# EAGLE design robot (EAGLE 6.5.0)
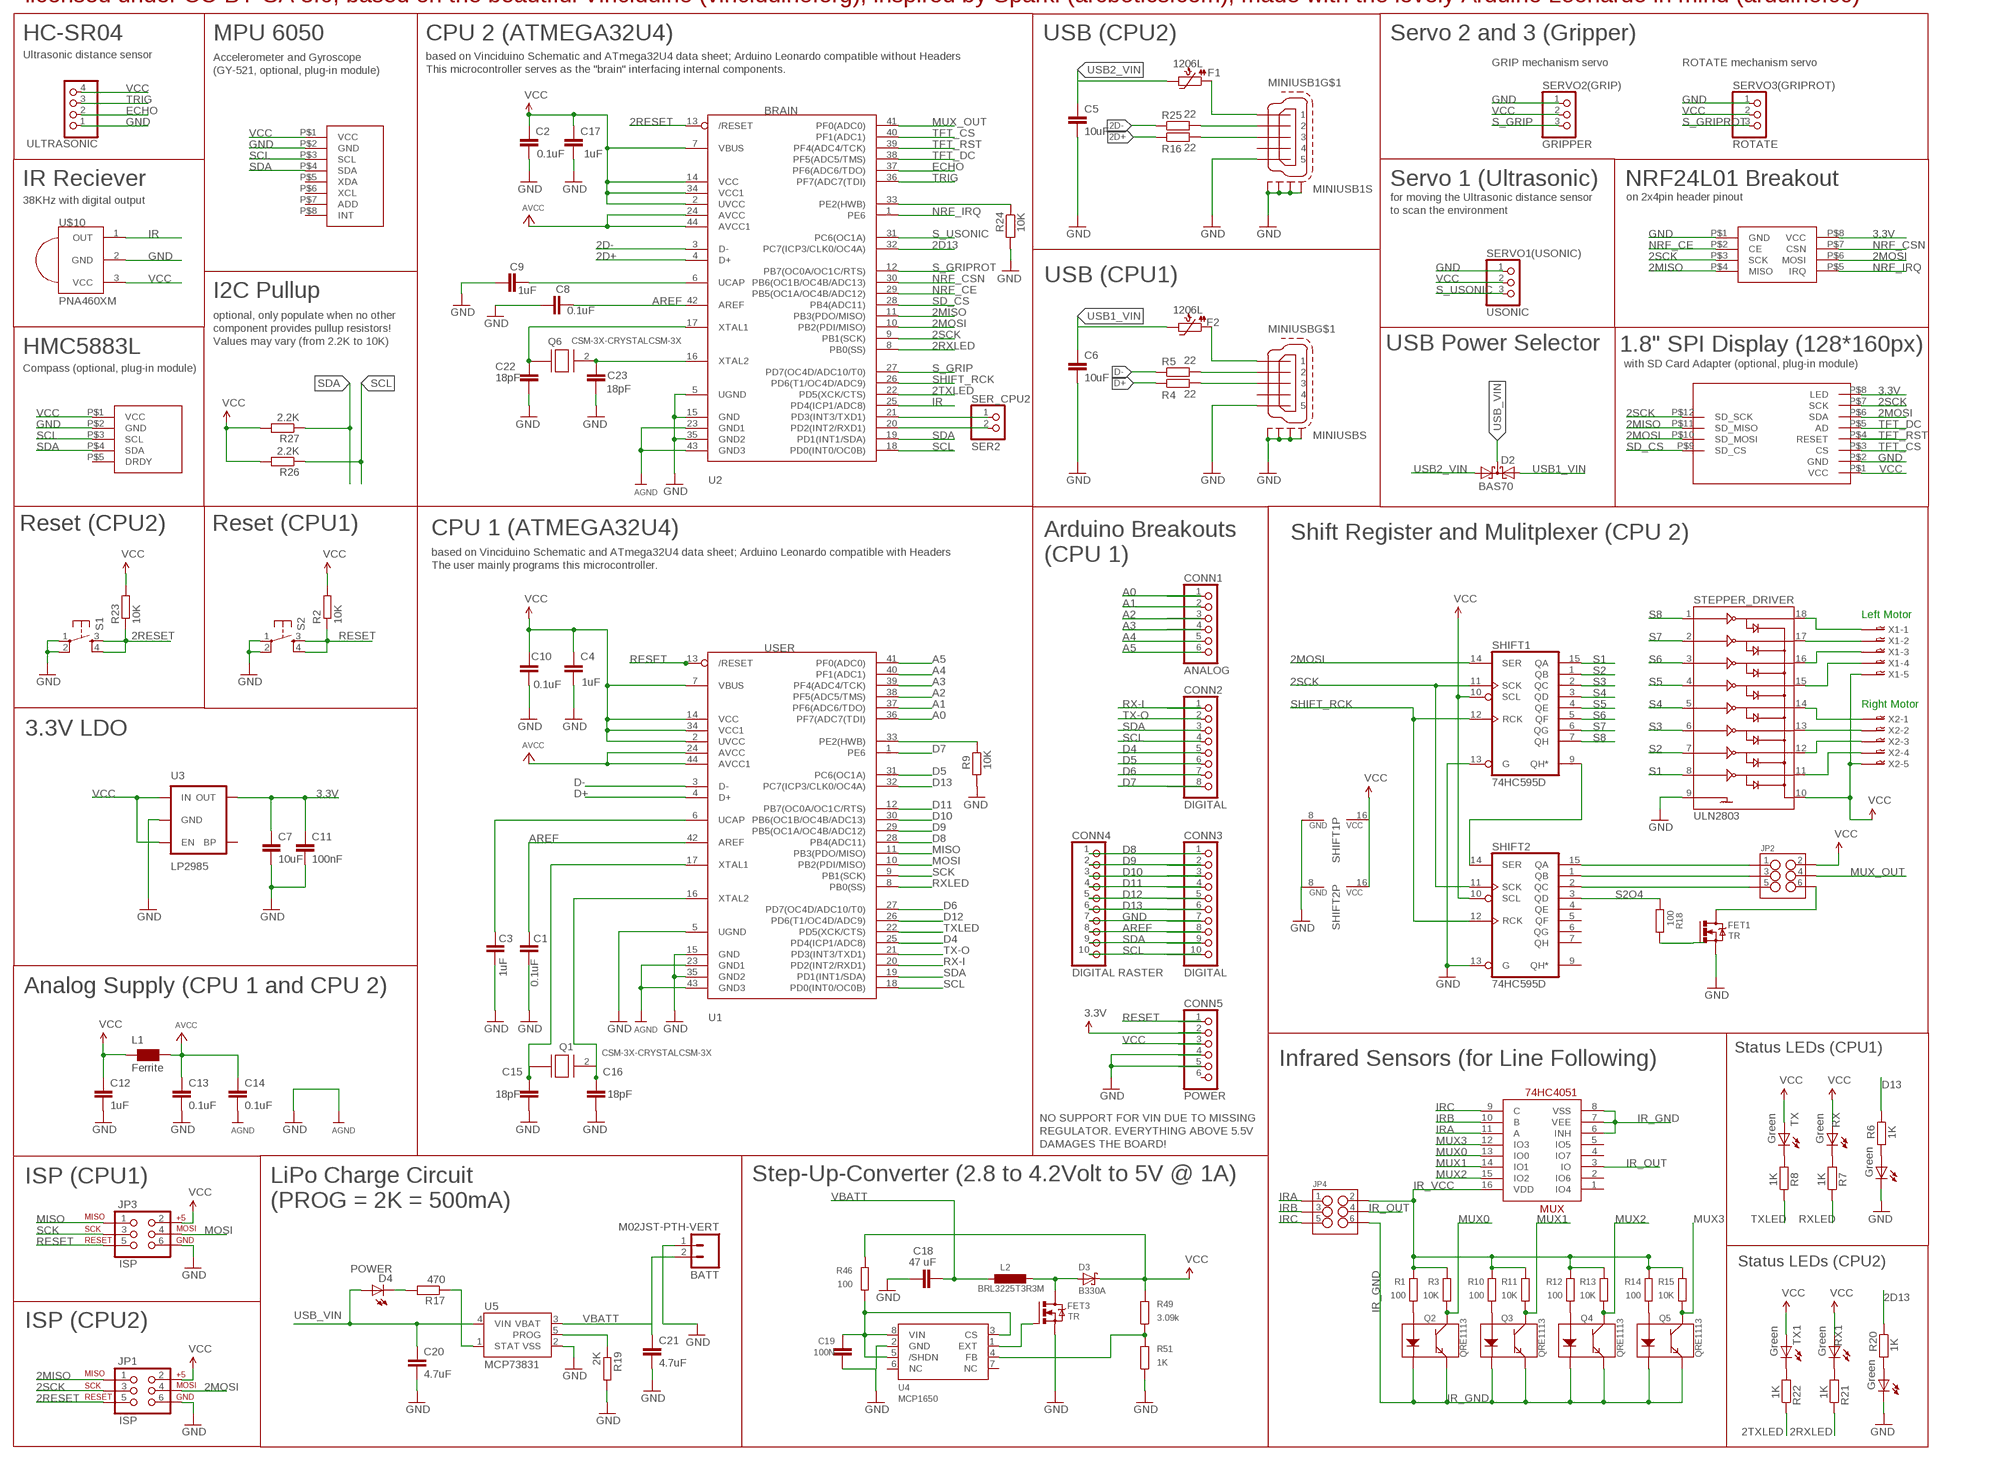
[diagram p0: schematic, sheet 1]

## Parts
BATT  M02JST-PTH-VERT  [JST-2-PTH-VERT]
C1  0.1uF  C-EUC1206  [C1206]
C2  0.1uF  C-EUC1206  [C1206]
C3  1uF  C-EUC1206  [C1206]
C4  1uF  C-EUC1206  [C1206]
C5  10uF  C-EUC1206  [C1206]
C6  10uF  C-EUC1206  [C1206]
C7  10uF  C-EUC1206  [C1206]
C8  0.1uF  C-EUC1206  [C1206]
C9  1uF  C-EUC1206  [C1206]
C10  0.1uF  C-EUC1206  [C1206]
C11  100nF  C-EUC1206  [C1206]
C12  1uF  C-EUC1206  [C1206]
C13  0.1uF  C-EUC1206  [C1206]
C14  0.1uF  C-EUC1206  [C1206]
C15  18pF  C-EUC1206  [C1206]
C16  18pF  C-EUC1206  [C1206]
C17  1uF  C-EUC1206  [C1206]
C18  47 uF  C-EUC1206  [C1206]
C19  100N  C-EUC1206  [C1206]
C20  4.7uF  C-EUC1206  [C1206]
C21  4.7uF  C-EUC1206  [C1206]
C22  18pF  C-EUC1206  [C1206]
C23  18pF  C-EUC1206  [C1206]
CONN1  ANALOG  PINHD-1X6B  [1X06-BIG]
CONN2  DIGITAL  PINHD-1X8BIG  [1X08-BIG]
CONN3  DIGITAL  PINHD-1X10  [1X10-BIG]
CONN4  DIGITAL RASTER  PINHD-1X10  [1X10-BIG]
CONN5  POWER  PINHD-1X6B  [1X06-BIG]
D2  BAS70  BAS70-05  [SOT23]
D3  B330A  [SMA]
D4  POWER  LED1206  [LED-1206]
D13  Green  LED1206  [LED-1206]
D13_2  Green  LED1206  [LED-1206]
F1  1206L  PTC1206_L  [1206_PTC]
F2  1206L  PTC1206_L  [1206_PTC]
FET1  TR  IRLML2502TR  [MICRO3]
FET3  TR  IRLML2502TR  [MICRO3]
JP1  ISP  AVR_SPI_PRG_6PTH  [2X3]
JP2  M03X22X3_SILK_SM  [2X3]
JP3  ISP  AVR_SPI_PRG_6PTH  [2X3]
JP4  M03X22X3_SILK_SM  [2X3]
L1  Ferrite  WE-CBF_1206W  [1206W]
L2  BRL3225T3R3M  L-EUL3225P  [L3225P]
MINIUSB  MINI-USB-SCHIELD-32005-201  [32005-201]
MINIUSB1  MINI-USB-SCHIELD-32005-201  [32005-201]
MUX  74HC4051  74HC4051_MUX  [SO16]
Q1  CSM-3X-CRYSTALCSM-3X  [CSM-3X]
Q2  QRE1113  [QRE1113]
Q3  QRE1113  [QRE1113]
Q4  QRE1113  [QRE1113]
Q5  QRE1113  [QRE1113]
Q6  CSM-3X-CRYSTALCSM-3X  [CSM-3X]
R1  100  R-EU_R1206  [R1206]
R2  10K  R-EU_R1206  [R1206]
R3  10K  R-EU_R1206  [R1206]
R4  22  R-EU_R1206  [R1206]
R5  22  R-EU_R1206  [R1206]
R6  1K  R-EU_R1206  [R1206]
R7  1K  R-EU_R1206  [R1206]
R8  1K  R-EU_R1206  [R1206]
R9  10K  R-EU_R1206  [R1206]
R10  100  R-EU_R1206  [R1206]
R11  10K  R-EU_R1206  [R1206]
R12  100  R-EU_R1206  [R1206]
R13  10K  R-EU_R1206  [R1206]
R14  100  R-EU_R1206  [R1206]
R15  10K  R-EU_R1206  [R1206]
R16  22  R-EU_R1206  [R1206]
R17  470  R-EU_R1206  [R1206]
R18  100  R-EU_R1206  [R1206]
R19  2K  R-EU_R1206  [R1206]
R20  1K  R-EU_R1206  [R1206]
R21  1K  R-EU_R1206  [R1206]
R22  1K  R-EU_R1206  [R1206]
R23  10K  R-EU_R1206  [R1206]
R24  10K  R-EU_R1206  [R1206]
R25  22  R-EU_R1206  [R1206]
R26  2.2K  R-EU_R1206  [R1206]
R27  2.2K  R-EU_R1206  [R1206]
R46  100  R-EU_R1206  [R1206]
R49  3.09k  R-EU_R1206  [R1206]
R51  1K  R-EU_R1206  [R1206]
RX  Green  LED1206  [LED-1206]
RX1  Green  LED1206  [LED-1206]
S1  Reset  TAC_SWITCHSMD  [TACTILE_SWITCH_SMD]
S2  Reset  TAC_SWITCHSMD  [TACTILE_SWITCH_SMD]
SER_CPU2  SER2  PINHD-1X2  [1X02]
SERVO1(USONIC)  USONIC  PINHD-1X3  [1X03]
SERVO2(GRIP)  GRIPPER  PINHD-1X3  [1X03]
SERVO3(GRIPROT)  ROTATE  PINHD-1X3  [1X03]
SHIFT1  74HC595D  [SO16]
SHIFT2  74HC595D  [SO16]
STEPPER_DRIVER  ULN2803  ULN2803SOIC  [SO018]
TX  Green  LED1206  [LED-1206]
TX1  Green  LED1206  [LED-1206]
U1  USER  ATMEGA32U4-AU  [TQFP44]
U2  BRAIN  ATMEGA32U4-AU  [TQFP44]
U3  LP2985  V_REG_LDOSMD  [SOT23-5@1]
U4  MCP1650  [MSOP8]
U5  MCP73831  MCP73831SMD  [SOT23-5]
U$2  1.8TFT+SD  [1.8TFTSD]
U$3  GY-521  [GY-521]
U$4  HMC5883L  [HMC5883L]
U$5  NRF24L01+  [NRF24L01+]
U$10  PNA460XM  [PNA460XM]
ULTRASONIC  PINHD-1X4  [1X04]
X1  05-JST-B5B-XH-A  [B5B-XH]
X2  05-JST-B5B-XH-A  [B5B-XH]

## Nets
2D13: R20.1 U2.32(PC7(ICP3/CLK0/OC4A))
2D+: R16.1 U2.4(D+)
2D-: R25.1 U2.3(D-)
2MISO: JP1.1 U2.11(PB3(PDO/MISO)) U$2.P$11(SD_MISO) U$5.P$4(MISO)
2MOSI: JP1.4 SHIFT1.14(SER) U2.10(PB2(PDI/MISO)) U$2.P$6(SDA) U$2.P$10(SD_MOSI) U$5.P$6(MOSI)
2RESET: JP1.5 R23.1 S1.3 S1.4 U2.13(/RESET)
2RXLED: R21.1 U2.8(PB0(SS))
2SCK: JP1.3 SHIFT1.11(SCK) SHIFT2.11(SCK) U2.9(PB1(SCK)) U$2.P$7(SCK) U$2.P$12(SD_SCK) U$5.P$3(SCK)
2TXLED: R22.1 U2.22(PD5(XCK/CTS))
2XTAL1: C22.1 Q6.1 U2.17(XTAL1)
2XTAL2: C23.1 Q6.2 U2.16(XTAL2)
3.3V: C7.1 C11.1 CONN5.2 U3.5(OUT) U$2.P$8(LED) U$5.P$8(VCC)
A0: CONN1.1 U1.36(PF7(ADC7(TDI))
A1: CONN1.2 U1.37(PF6(ADC6/TDO))
A2: CONN1.3 U1.38(PF5(ADC5/TMS))
A3: CONN1.4 U1.39(PF4(ADC4/TCK))
A4: CONN1.5 U1.40(PF1(ADC1))
A5: CONN1.6 U1.41(PF0(ADC0))
AREF: C1.2 C8.2 CONN3.8 CONN4.8 U1.42(AREF) U2.42(AREF)
AVCC: C13.1 C14.1 L1.2 U1.24(AVCC) U1.44(AVCC1) U2.24(AVCC) U2.44(AVCC1)
D4: CONN2.5 U1.25(PD4(ICP1/ADC8))
D5: CONN2.6 U1.31(PC6(OC1A))
D6: CONN2.7 U1.27(PD7(OC4D/ADC10/T0))
D7: CONN2.8 U1.1(PE6)
D8: CONN3.1 CONN4.1 U1.28(PB4(ADC11))
D9: CONN3.2 CONN4.2 U1.29(PB5(OC1A/OC4B/ADC12))
D10: CONN3.3 CONN4.3 U1.30(PB6(OC1B/OC4B/ADC13))
D11: CONN3.4 CONN4.4 U1.12(PB7(OC0A/OC1C/RTS))
D12: CONN3.5 CONN4.5 U1.26(PD6(T1/OC4D/ADC9))
D13: CONN3.6 CONN4.6 R6.1 U1.32(PC7(ICP3/CLK0/OC4A))
D+: R4.1 U1.4(D+)
D-: R5.1 U1.3(D-)
ECHO: U2.37(PF6(ADC6/TDO)) ULTRASONIC.2
GND: BATT.1 C1.1 C2.2 C3.2 C4.2 C5.2 C6.2 C7.2 C8.1 C9.2 C10.2 C11.2 C12.2 C13.2 C14.2 C15.2 C16.2 C17.2 C18.1 C19.2 C20.2 C21.2 C22.2 C23.2 CONN3.7 CONN4.7 CONN5.4 CONN5.5 D13.C D13_2.C FET1.2(S) FET3.2(S) JP1.6 JP3.6 MINIUSB1.5 MINIUSB1.M1(S:S1) MINIUSB1.M2(S:S2) MINIUSB1.M3(S:S3) MINIUSB1.M4(S:S4) MINIUSB.5 MINIUSB.M1(S:S1) MINIUSB.M2(S:S2) MINIUSB.M3(S:S3) MINIUSB.M4(S:S4) R9.2 R19.2 R24.2 R51.1 S1.1 S1.2 S2.1 S2.2 SERVO1(USONIC).1 SERVO2(GRIP).1 SERVO3(GRIPROT).1 SHIFT1.8(GND) SHIFT1.13(G) SHIFT2.8(GND) SHIFT2.13(G) STEPPER_DRIVER.9 U1.5(UGND) U1.15(GND) U1.23(GND1) U1.35(GND2) U1.43(GND3) U2.5(UGND) U2.15(GND) U2.23(GND1) U2.35(GND2) U2.43(GND3) U3.2(GND) U4.2(GND) U5.2(VSS) U$2.P$2(GND) U$3.P$2(GND) U$4.P$2(GND) U$5.P$1(GND) U$10.2(GND) ULTRASONIC.1 ; supply symbol labelled AGND
IR: U2.25(PD4(ICP1/ADC8)) U$10.1(OUT)
IR_GND: JP4.6 MUX.6(INH) MUX.7(VEE) MUX.8(VSS) Q2.2(K) Q2.4(E) Q3.2(K) Q3.4(E) Q4.2(K) Q4.4(E) Q5.2(K) Q5.4(E)
IR_OUT: JP4.4 MUX.3(IO)
IR_VCC: JP4.2 MUX.16(VDD) R1.2 R3.2 R10.2 R11.2 R12.2 R13.2 R14.2 R15.2
IRA: JP4.1 MUX.11(A)
IRB: JP4.3 MUX.10(B)
IRC: JP4.5 MUX.9(C)
MISO: JP3.1 U1.11(PB3(PDO/MISO))
MOSI: JP3.4 U1.10(PB2(PDI/MISO))
MUX0: MUX.13(IO0) Q2.3(C) R3.1
MUX1: MUX.14(IO1) Q3.3(C) R11.1
MUX2: MUX.15(IO2) Q4.3(C) R13.1
MUX3: MUX.12(IO3) Q5.3(C) R15.1
MUX_OUT: JP2.4 U2.41(PF0(ADC0))
N$1: R8.2 TX.C
N$2: MINIUSB.2 R5.2
N$3: SER_CPU2.1 U2.21(PD3(INT3/TXD1))
N$4: SER_CPU2.2 U2.20(PD2(INT2/RXD1))
N$5: MINIUSB.3 R4.2
N$6: R9.1 U1.33(PE2(HWB))
N$7: D13.A R6.2
N$8: C9.1 U2.6(UCAP)
N$9: R7.2 RX.C
N$10: Q2.1(A) R1.1
N$11: Q3.1(A) R10.1
N$12: Q4.1(A) R12.1
N$13: F2.1 MINIUSB.1
N$14: Q5.1(A) R14.1
N$15: C3.1 U1.6(UCAP)
N$16: FET1.1(G) R18.2
N$17: R24.1 U2.33(PE2(HWB))
N$18: F1.1 MINIUSB1.1
N$19: FET3.1(G) U4.1(EXT)
N$20: R19.1 U5.5(PROG)
N$21: R17.1 U5.1(STAT)
N$22: D4.C R17.2
N$23: R49.1 R51.2 U4.4(FB)
N$24: D3.A FET3.3(D) L2.2
N$25: C19.1 R46.1 U4.3(CS) U4.5(/SHDN) U4.8(VIN)
N$26: STEPPER_DRIVER.11 X2.P$4
N$27: STEPPER_DRIVER.12 X2.P$3
N$28: STEPPER_DRIVER.13 X2.P$2
N$29: STEPPER_DRIVER.14 X2.P$1
N$30: STEPPER_DRIVER.15 X1.P$4
N$31: STEPPER_DRIVER.16 X1.P$3
N$32: STEPPER_DRIVER.17 X1.P$2
N$33: STEPPER_DRIVER.18 X1.P$1
N$34: D13_2.A R20.2
N$35: R22.2 TX1.C
N$36: R21.2 RX1.C
N$37: MINIUSB1.2 R25.2
N$38: MINIUSB1.3 R16.2
N$41: JP2.1 SHIFT2.15(QA)
N$42: JP2.3 SHIFT2.1(QB)
N$43: JP2.5 SHIFT2.2(QC)
N$45: FET1.3(D) JP2.6
NRF_CE: U2.29(PB5(OC1A/OC4B/ADC12)) U$5.P$2(CE)
NRF_CSN: U2.30(PB6(OC1B/OC4B/ADC13)) U$5.P$7(CSN)
NRF_IRQ: U2.1(PE6) U$5.P$5(IRQ)
RESET: CONN5.1 JP3.5 R2.1 S2.3 S2.4 U1.13(/RESET)
RX-I: CONN2.1 U1.20(PD2(INT2/RXD1))
RXLED: R7.1 U1.8(PB0(SS))
S1: SHIFT1.15(QA) STEPPER_DRIVER.8
S1OVERFLOW: SHIFT1.9(QH*) SHIFT2.14(SER)
S2: SHIFT1.1(QB) STEPPER_DRIVER.7
S2O4: R18.1 SHIFT2.3(QD)
S3: SHIFT1.2(QC) STEPPER_DRIVER.6
S4: SHIFT1.3(QD) STEPPER_DRIVER.5
S5: SHIFT1.4(QE) STEPPER_DRIVER.4
S6: SHIFT1.5(QF) STEPPER_DRIVER.3
S7: SHIFT1.6(QG) STEPPER_DRIVER.2
S8: SHIFT1.7(QH) STEPPER_DRIVER.1
S_GRIP: SERVO2(GRIP).3 U2.27(PD7(OC4D/ADC10/T0))
S_GRIPROT: SERVO3(GRIPROT).3 U2.12(PB7(OC0A/OC1C/RTS))
S_USONIC: SERVO1(USONIC).3 U2.31(PC6(OC1A))
SCK: JP3.3 U1.9(PB1(SCK))
SCL: CONN2.4 CONN3.10 CONN4.10 R26.1 U1.18(PD0(INT0/OC0B)) U2.18(PD0(INT0/OC0B)) U$3.P$3(SCL) U$4.P$3(SCL)
SD_CS: U2.28(PB4(ADC11)) U$2.P$9(SD_CS)
SDA: CONN2.3 CONN3.9 CONN4.9 R27.1 U1.19(PD1(INT1/SDA)) U2.19(PD1(INT1/SDA)) U$3.P$4(SDA) U$4.P$4(SDA)
SHIFT_RCK: SHIFT1.12(RCK) SHIFT2.12(RCK) U2.26(PD6(T1/OC4D/ADC9))
TFT_CS: U2.40(PF1(ADC1)) U$2.P$3(CS)
TFT_DC: U2.38(PF5(ADC5/TMS)) U$2.P$5(AD)
TFT_RST: U2.39(PF4(ADC4/TCK)) U$2.P$4(RESET)
TRIG: U2.36(PF7(ADC7(TDI)) ULTRASONIC.3
TX-O: CONN2.2 U1.21(PD3(INT3/TXD1))
TXLED: R8.1 U1.22(PD5(XCK/CTS))
USB1_VIN: C6.1 D2.2(A2) F2.2
USB2_VIN: C5.1 D2.1(A1) F1.2
USB_VIN: C20.1 D2.3(C) D4.A U5.4(VIN)
VBATT: BATT.2 C18.2 C21.1 L2.1 U5.3(VBAT)
VCC: C2.1 C4.1 C10.1 C12.1 C17.1 CONN5.3 D3.C JP1.2 JP2.2 JP3.2 L1.1 R2.2 R23.2 R26.2 R27.2 R46.2 R49.2 RX1.A RX.A SERVO1(USONIC).2 SERVO2(GRIP).2 SERVO3(GRIPROT).2 SHIFT1.10(SCL) SHIFT1.16(VCC) SHIFT2.10(SCL) SHIFT2.16(VCC) STEPPER_DRIVER.10 TX1.A TX.A U1.2(UVCC) U1.7(VBUS) U1.14(VCC) U1.34(VCC1) U2.2(UVCC) U2.7(VBUS) U2.14(VCC) U2.34(VCC1) U3.1(IN) U3.3(EN) U$2.P$1(VCC) U$3.P$1(VCC) U$4.P$1(VCC) U$10.3(VCC) ULTRASONIC.4 X1.P$5 X2.P$5
XTAL1: C15.1 Q1.1 U1.17(XTAL1)
XTAL2: C16.1 Q1.2 U1.16(XTAL2)
Unconnected: CONN5.6 MINIUSB1.4 MINIUSB.4 MUX.1(IO4) MUX.2(IO6) MUX.4(IO7) MUX.5(IO5) SHIFT2.4(QE) SHIFT2.5(QF) SHIFT2.6(QG) SHIFT2.7(QH) SHIFT2.9(QH*) U3.4(BP) U4.6(NC) U4.7(NC) U$3.P$5(XDA) U$3.P$6(XCL) U$3.P$7(ADD) U$3.P$8(INT) U$4.P$5(DRDY)

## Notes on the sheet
- Edubot V.0.1 by Sebastian Muszytowski <muzy@chaosdorf.de>
- licensed under CC-BY-SA 3.0, based on the beautiful Vinciduino (vinciduino.org), inspired by Sparki (arcbotics.com), made with the lovely Arduino Leonardo in mind (arduino.cc)
- HC-SR04 | MPU 6050 | CPU 2 (ATMEGA32U4) | USB (CPU2) | Servo 2 and 3 (Gripper)
- Ultrasonic distance sensor
- GRIP mechanism servo | ROTATE mechanism servo
- based on Vinciduino Schematic and ATmega32U4 data sheet; Arduino Leonardo compatible without Headers
  This microcontroller serves as the "brain" interfacing internal components.
- Accelerometer and Gyroscope 
  (GY-521, optional, plug-in module)
- IR Reciever | Servo 1 (Ultrasonic) | NRF24L01 Breakout
- on 2x4pin header pinout
- 38KHz with digital output
- for moving the Ultrasonic distance sensor
  to scan the environment
- USB (CPU1)
- I2C Pullup
- optional, only populate when no other
  component provides pullup resistors!
  Values may vary (from 2.2K to 10K)
- HMC5883L | USB Power Selector | 1.8" SPI Display (128*160px)
- with SD Card Adapter (optional, plug-in module)
- Compass (optional, plug-in module)
- Reset (CPU2) | Reset (CPU1) | CPU 1 (ATMEGA32U4)
- Shift Register and Mulitplexer (CPU 2)
- Arduino Breakouts
  (CPU 1)
- based on Vinciduino Schematic and ATmega32U4 data sheet; Arduino Leonardo compatible with Headers
  The user mainly programs this microcontroller.
- Left Motor
- Right Motor
- 3.3V LDO
- Analog Supply (CPU 1 and CPU 2)
- Status LEDs (CPU1)
- Infrared Sensors (for Line Following)
- NO SUPPORT FOR VIN DUE TO MISSING
  REGULATOR. EVERYTHING ABOVE 5.5V
  DAMAGES THE BOARD!
- ISP (CPU1) | Step-Up-Converter (2.8 to 4.2Volt to 5V @ 1A)
- LiPo Charge Circuit
  (PROG = 2K = 500mA)
- Status LEDs (CPU2)
- ISP (CPU2)

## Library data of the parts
BATT = SparkFun-Connectors:M02: Standard 2-pin 0.1" header. Use with
C1-C23 = resistor:C-EU: CAPACITOR, European symbol
CONN1 CONN5 = adafruit:PINHD-1X6: PIN HEADER
CONN2 = adafruit:PINHD-1X8: PIN HEADER
CONN3 CONN4 = adafruit:PINHD-1X10: Pin header 1x10 0.1" spacing With round pins
D2 = diode:BAS70-05: Silicon Schottky Diodes General-purpose diode for high-speed switching
D3 = aaron_discrete:B330A: SCHOTTKY DIODE
D4 D13 D13_2 RX RX1 TX TX1 = SparkFun-LED:LED: LEDs
F1 F2 = microbuilder:PTC: PTC (Resettable Fuse)
FET1 FET3 = aaron_discrete:IRLML2502TR
JP1 JP3 = SparkFun:AVR_SPI_PRG_6: AVR ISP 6 Pin This is the reduced ISP connector for AVR programming. Common on Arduino. This footprint will take up less PCB space and can be used with a 10-pin to 6-pin adapter such as SKU: BOB-08508
JP2 JP4 = SparkFun-Connectors:M03X2: 2x3 .1" header. Shrouded, with keying- CONN-10681 SMT- CONN-11415 Pogo pins- HW-11044
L1 = wuerth-elektronik:WE-CBF: SMD EMI Suppression Ferrite Beads
L2 = resistor:L-EU: INDUCTOR, European symbol
MINIUSB MINIUSB1 = con-cypressindustries:MINI-USB-SCHIELD-: MINI USB-B Conector Source: www.cypressindustries.com; OC_FARNELL: unknown; OC_NEWARK: unknown
MUX = SparkFun-AnalogIC:74HC4051_MUX: 8:1 analog mux
Q1 Q6 = fmc:CSM-3X-CRYSTAL
Q2-Q5 = aaron_discrete:QRE1113: Surface-mount IR reflective sensor - 5mm range
R1-R27 R46 R49 R51 = resistor:R-EU_: RESISTOR, European symbol
S1 S2 = SparkFun:TAC_SWITCH: Momentary Switch Button commonly used for reset or general input. Spark Fun Electronics SKU : COM-00097
SER_CPU2 = pinhead:PINHD-1X2: PIN HEADER
SERVO1(USONIC) SERVO2(GRIP) SERVO3(GRIPROT) = pinhead:PINHD-1X3: PIN HEADER
SHIFT1 SHIFT2 = 74xx-eu:74*595: 8-bit SHIFT REGISTER, output latch
STEPPER_DRIVER = SparkFun-PowerIC:ULN2803: Darlington Driver ULN2803 Darlington array. 500mA max per channel, 8-channel package. Spark Fun Electronics SKU : COM-00312
U1 U2 = adafruit:ATMEGA32U4: http://www.ladyada.net/library/eagle
U3 = SparkFun:V_REG_LDO: Voltage Regulator LDO Standard 150mA LDO voltage regulator in SOT-23 layout. Micrel part MIC5205. BP (by-pass) pin is used to lower output noise with 470pF cap.
U4 = aaron_ic:MCP1650: IC CONTROLLER BOOST 2.55V 8MSOP
U5 = SparkFun:MCP73831
U$2 = muzy_robot:1.8TFT+SD: 1.8" FT + SD Card Reader
U$3 = muzy_robot:GY-521: GY-521 Accelerometer and Gyroscope
U$4 = muzy_robot:HMC5883L: HMC5883L compass module
U$5 = muzy_robot:NRF24L01+: NRF24L01+ module
U$10 = adafruit:PNA460XM: IR 38KHz receiver PNA4602 and related receivers http://www.ladyada.net/library/pcb/eaglelibrary.html
ULTRASONIC = pinhead:PINHD-1X4: PIN HEADER
X1 X2 = con-jst-xh:05-JST: JST CONNECTOR

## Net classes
1 vcc: width 0.254 mm

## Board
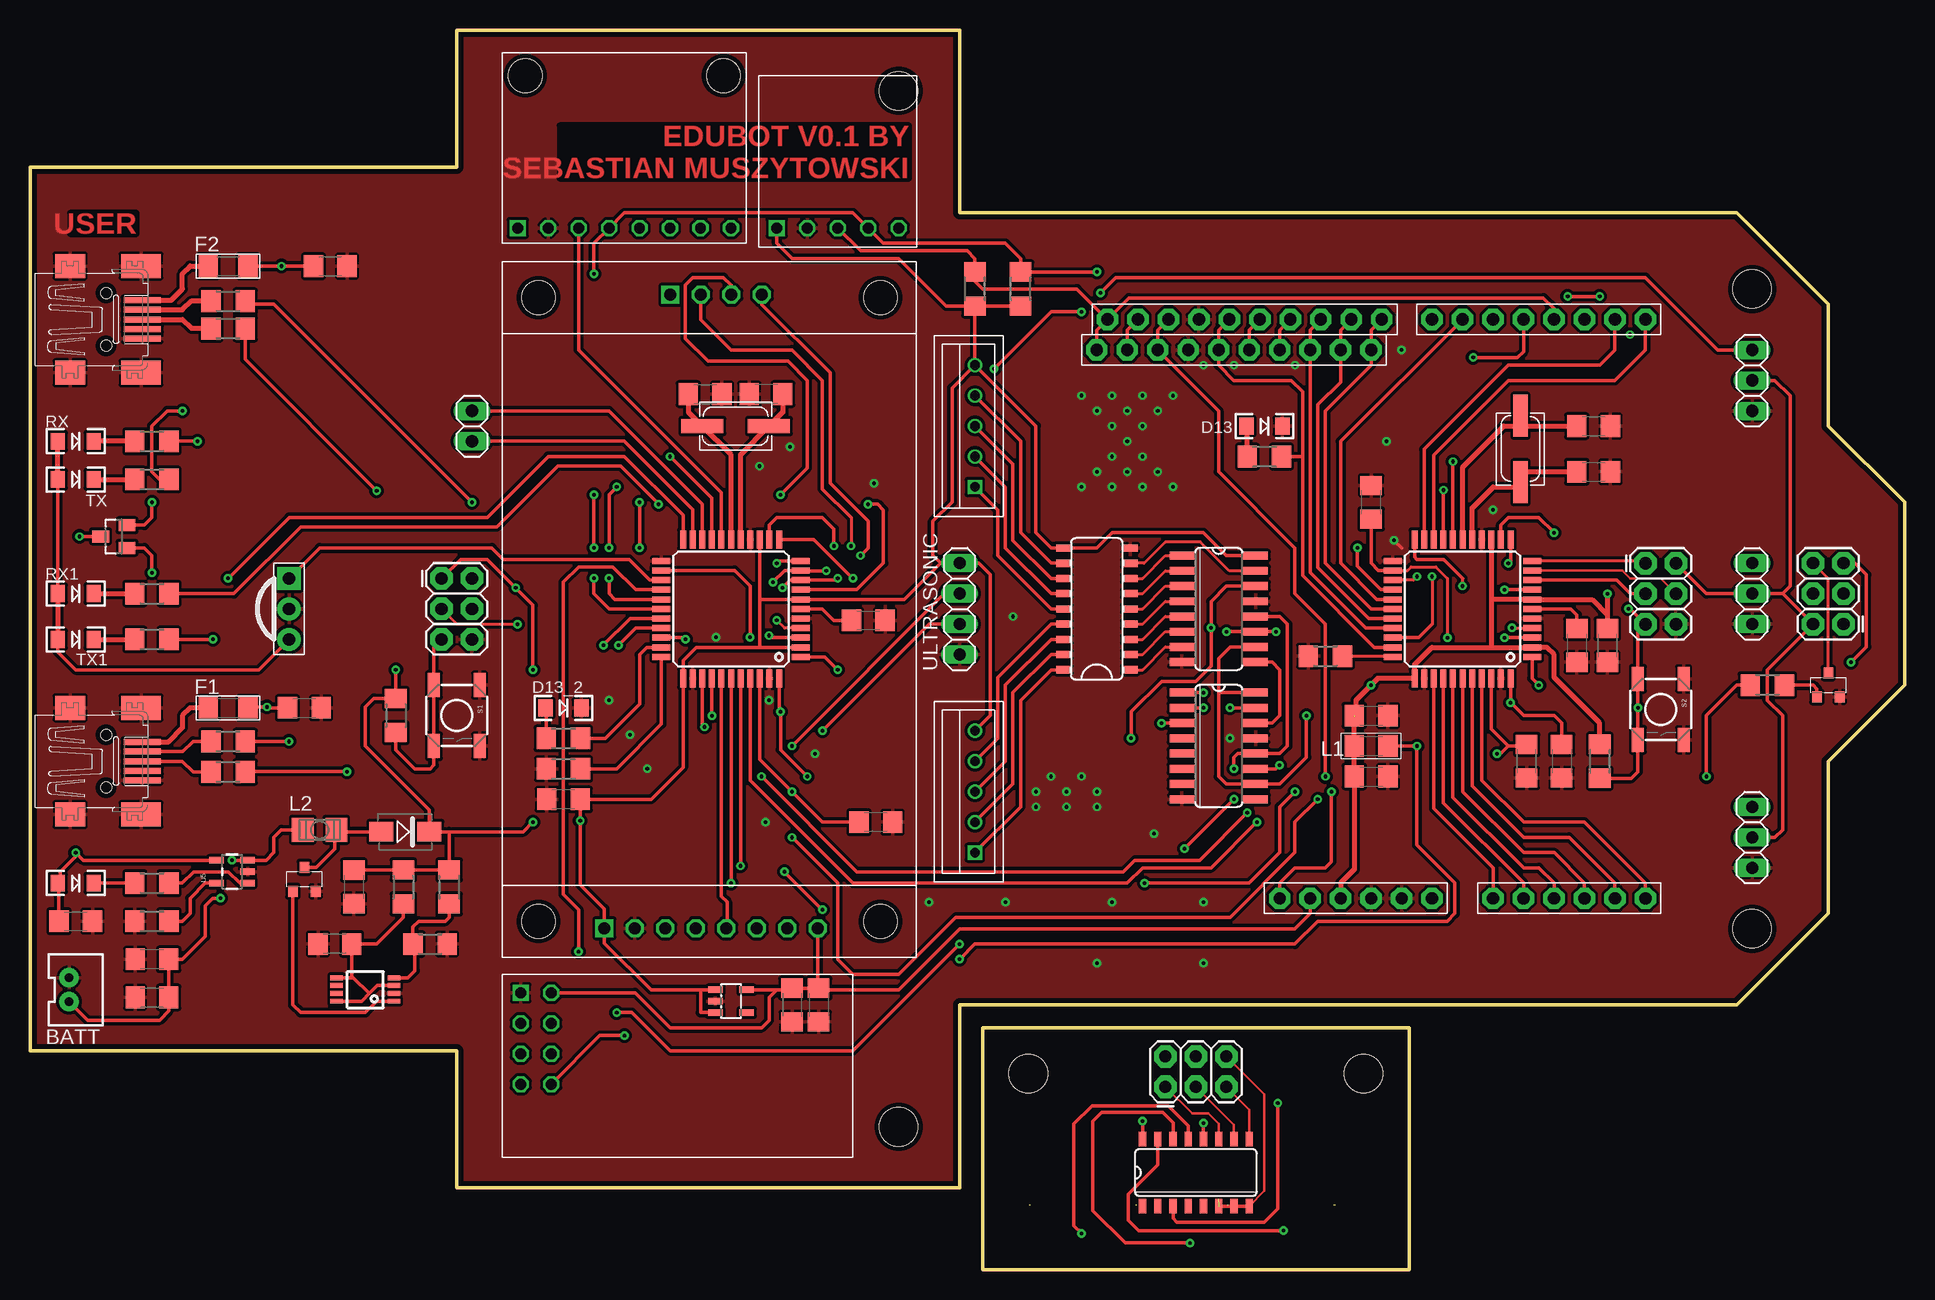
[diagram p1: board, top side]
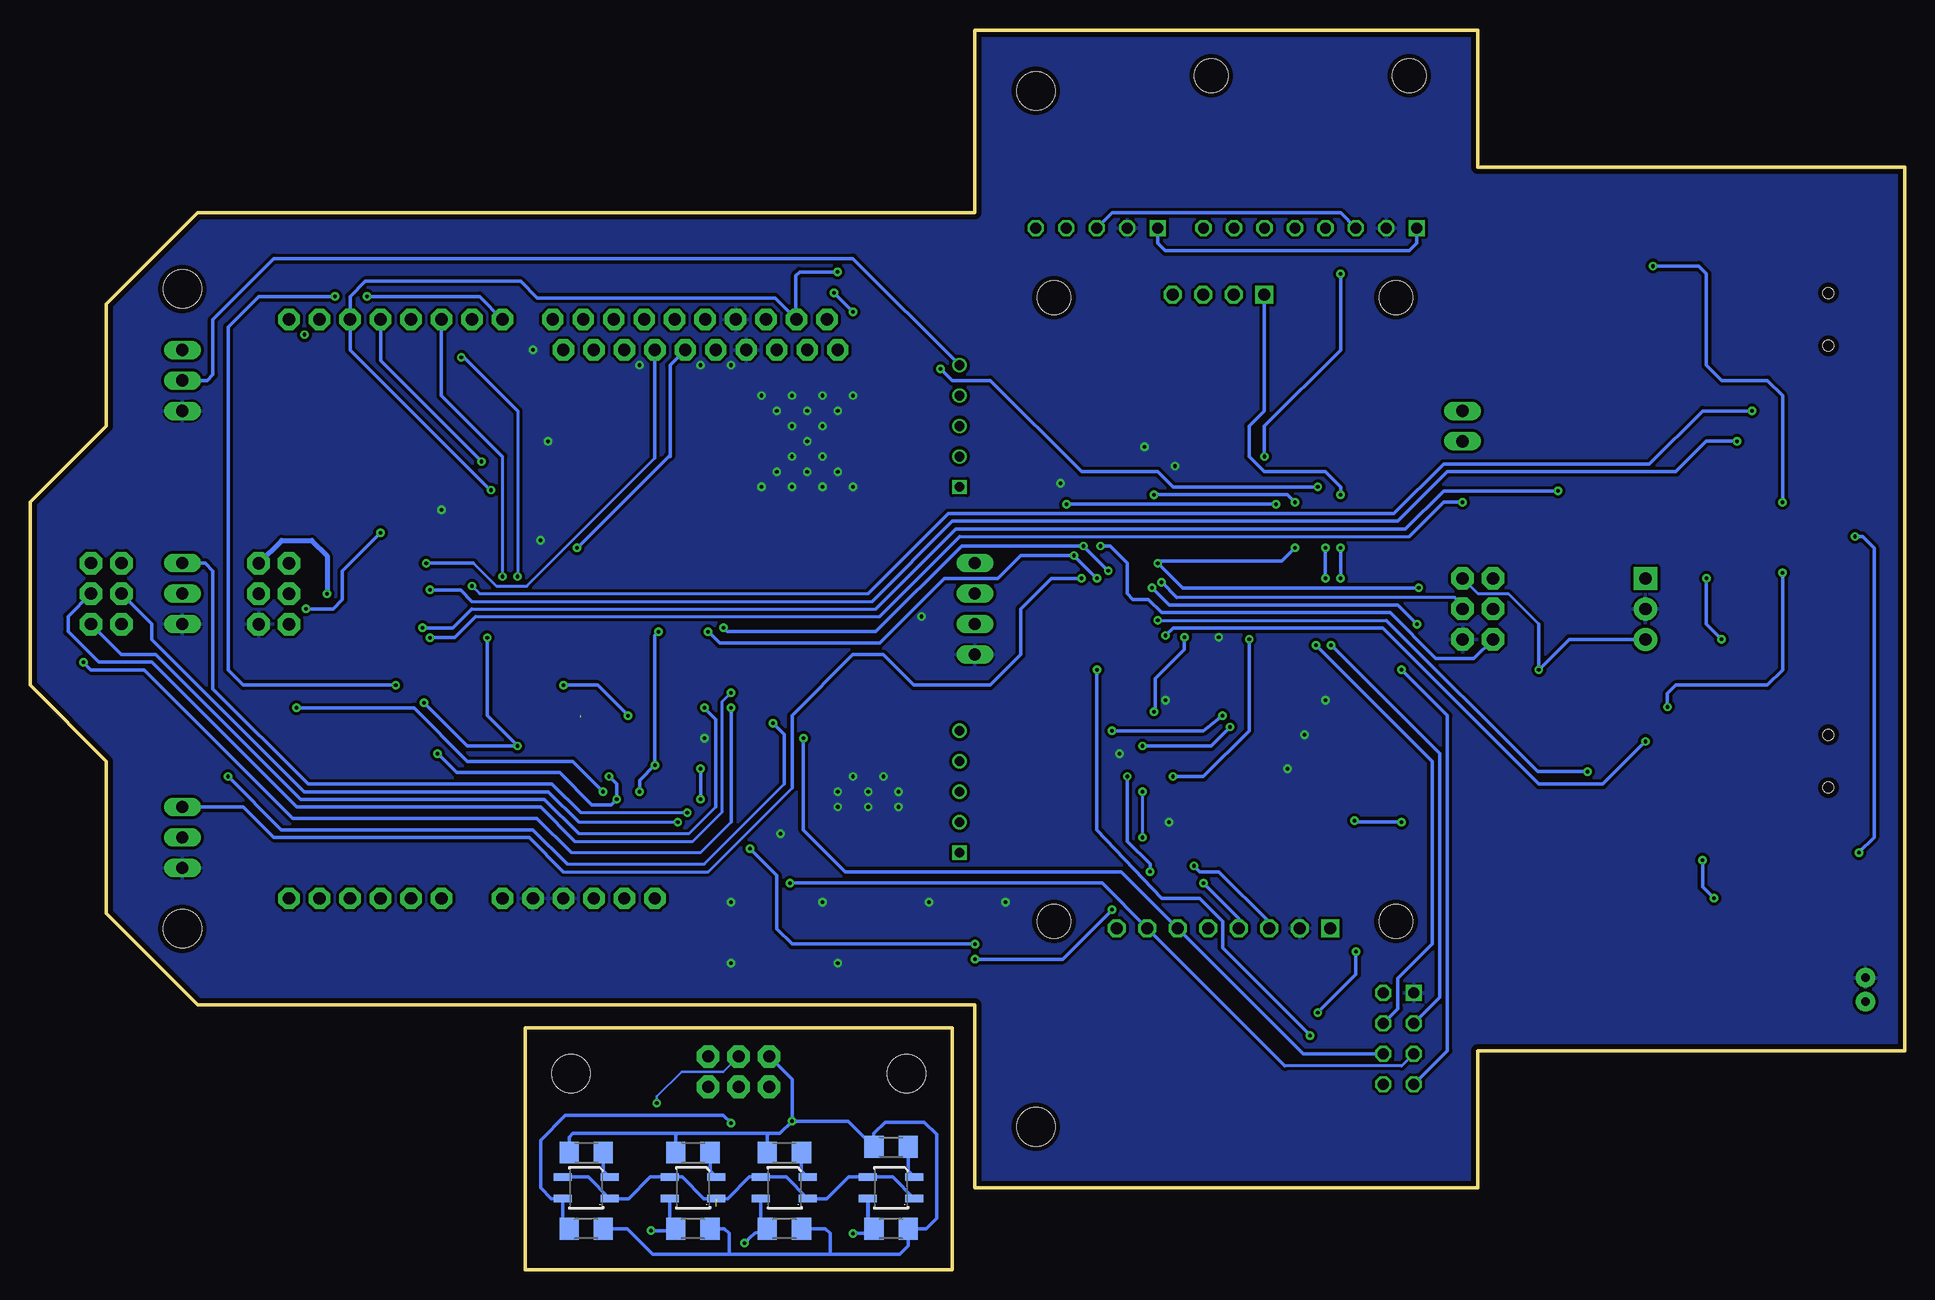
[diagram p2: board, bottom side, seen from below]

Size 156.21 x 103.35 mm. Coordinates in mm from the lower left corner, seen from the top.
Outline: 79.38,20.16 114.94,20.16 114.94,0 79.38,0 79.38,20.16
Outline: 156.21,48.74 149.86,42.39 149.86,29.69 142.24,22.07 77.47,22.07 77.47,6.83 35.56,6.83 35.56,18.26 0,18.26 0,91.92 35.56,91.92 35.56,103.35 77.47,103.35 77.47,88.11 142.24,88.11 149.86,80.49 149.86,70.33 156.21,63.98 156.21,48.74
Copper layers (1*16): Top 0.035mm / dielectric 1.5mm / Bottom 0.035mm
Design rules "pcb-devboards_35µmCU_200µm_Strukturen_Abstaende": minimum track width 0.2mm, minimum drill 0.3mm, track to track 0.2mm, track to pad 0.2mm, pad to pad 0.2mm, via to via 0.2mm, smd to smd 0.2mm, copper to edge 0.4mm, drill to drill 0.4mm, minimum pad ring 0.2mm, minimum via ring 0.2mm, stop-mask expansion 4mil, vias tented up to drill 0mil, thermal gap 0.2mm
Holes 3.2 mm at 83.19,16.35 111.12,16.35 72.39,11.91 72.39,98.27 143.51,81.76 143.51,28.42

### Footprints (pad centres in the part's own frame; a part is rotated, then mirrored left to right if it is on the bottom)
JST-2-PTH-VERT = drill 0.7 pad 1.626: 1 -1,-0.55; 2 1,-0.55
C1206 = smd 1.6 x 1.8: 1 -1.4,0; 2 1.4,0
1X06-BIG = drill 1.016 pad 1.778 octagon: 1 -6.35,0; 2 -3.81,0; 3 -1.27,0; 4 1.27,0; 5 3.81,0; 6 6.35,0
1X08-BIG = drill 1.016 pad 1.778 octagon: 1 -8.89,0; 2 -6.35,0; 3 -3.81,0; 4 -1.27,0; 5 1.27,0; 6 3.81,0; 7 6.35,0; 8 8.89,0
1X10-BIG = drill 1.016 pad 1.778 octagon: 1 -11.43,0; 2 -8.89,0; 3 -6.35,0; 4 -3.81,0; 5 -1.27,0; 6 1.27,0; 7 3.81,0; 8 6.35,0; 9 8.89,0; 10 11.43,0
SOT23 = smd 1 x 1.4: 1 -0.95,-1.1; 2 0.95,-1.1; 3 0,1.1
SMA = smd 2 x 1.65: A 5,0.8; C 1,0.8
LED-1206 = smd 1.2 x 1.4: A -1.5,0; C 1.5,0
1206_PTC = smd 1.6 x 1.8: 1 -1.654,0; 2 1.654,0
MICRO3 = smd 0.8 x 0.9: 1 -0.95,-1; 2 0.95,-1; 3 0,1
2X3 = drill 1.016 pad 1.88 octagon: 1 0,0; 2 0,2.54; 3 2.54,0; 4 2.54,2.54; 5 5.08,0; 6 5.08,2.54
1206W = smd 1.6 x 1.8: 1 -1.4,0; 2 1.4,0
L3225P = smd 1.8 x 2: 1 -1.4,0; 2 1.4,0
32005-201 = smd 3.1 x 0.5: 1 3,1.6; 2 3,0.8; 3 3,0; 4 3,-0.8; 5 3,-1.6 | smd 2.5 x 2: M1 -3,-4.45; M2 -3,4.45 | smd 3.3 x 2: M3 2.9,4.45; M4 2.9,-4.45 | hole 0.9: 0,2.2; 0,-2.2
SO16 = smd 0.6 x 1.2: 1 -4.445,-2.8; 2 -3.175,-2.8; 3 -1.905,-2.8; 4 -0.635,-2.8; 5 0.635,-2.8; 6 1.905,-2.8; 7 3.175,-2.8; 8 4.445,-2.8; 9 4.445,2.8; 10 3.175,2.8; 11 1.905,2.8; 12 0.635,2.8; 13 -0.635,2.8; 14 -1.905,2.8; 15 -3.175,2.8; 16 -4.445,2.8
CSM-3X = smd 3.5 x 1.2: 1 2.775,0; 2 -2.775,0
QRE1113 = smd 1.5 x 0.6: 1 -1.95,-0.9; 2 1.95,-0.9; 3 1.95,0.9; 4 -1.95,0.9
R1206 = smd 1.6 x 1.803: 1 -1.422,0; 2 1.422,0
TACTILE_SWITCH_SMD = smd 2 x 1: 1 -2.54,1.905; 2 2.54,1.905; 3 -2.54,-1.905; 4 2.54,-1.905
1X02 = drill 1.016 long: 1 -1.27,0; 2 1.27,0
1X03 = drill 1.016 long: 1 -2.54,0; 2 0,0; 3 2.54,0
SO16' = smd 0.66 x 2.032: 1 -4.445,-3.073; 2 -3.175,-3.073; 3 -1.905,-3.073; 4 -0.635,-3.073; 5 0.635,-3.073; 6 1.905,-3.073; 7 3.175,-3.073; 8 4.445,-3.073; 9 4.445,3.073; 10 3.175,3.073; 11 1.905,3.073; 12 0.635,3.073; 13 -0.635,3.073; 14 -1.905,3.073; 15 -3.175,3.073; 16 -4.445,3.073
SO018 = smd 0.6 x 1.2: 1 -5.08,-2.8; 2 -3.81,-2.8; 3 -2.54,-2.8; 4 -1.27,-2.8; 5 0,-2.8; 6 1.27,-2.8; 7 2.54,-2.8; 8 3.81,-2.8; 9 5.08,-2.8; 10 5.08,2.8; 11 3.81,2.8; 12 2.54,2.8; 13 1.27,2.8; 14 0,2.8; 15 -1.27,2.8; 16 -2.54,2.8; 17 -3.81,2.8; 18 -5.08,2.8
TQFP44 = smd 1.5 x 0.5: 1 -5.8,4; 2 -5.8,3.2; 3 -5.8,2.4; 4 -5.8,1.6; 5 -5.8,0.8; 6 -5.8,0; 7 -5.8,-0.8; 8 -5.8,-1.6; 9 -5.8,-2.4; 10 -5.8,-3.2; 11 -5.8,-4; 23 5.8,-4; 24 5.8,-3.2; 25 5.8,-2.4; 26 5.8,-1.6; 27 5.8,-0.8; 28 5.8,0; 29 5.8,0.8; 30 5.8,1.6; 31 5.8,2.4; 32 5.8,3.2; 33 5.8,4 | smd 0.5 x 1.5: 12 -4,-5.8; 13 -3.2,-5.8; 14 -2.4,-5.8; 15 -1.6,-5.8; 16 -0.8,-5.8; 17 0,-5.8; 18 0.8,-5.8; 19 1.6,-5.8; 20 2.4,-5.8; 21 3.2,-5.8; 22 4,-5.8; 34 4,5.8; 35 3.2,5.8; 36 2.4,5.8; 37 1.6,5.8; 38 0.8,5.8; 39 0,5.8; 40 -0.8,5.8; 41 -1.6,5.8; 42 -2.4,5.8; 43 -3.2,5.8; 44 -4,5.8
SOT23-5@1 = smd 0.55 x 1.2: 1 -0.95,-1.3; 2 0,-1.3; 3 0.95,-1.3; 4 0.95,1.3; 5 -0.95,1.3
MSOP8 = smd 0.41 x 1.02: 1 -0.95,-2.4; 2 -0.3,-2.4; 3 0.35,-2.4; 4 1,-2.4; 5 1,2.4; 6 0.35,2.4; 7 -0.3,2.4; 8 -0.95,2.4
SOT23-5 = smd 0.55 x 1.2: 1 -0.95,-1.3; 2 0,-1.3; 3 0.95,-1.3; 4 0.95,1.3; 5 -0.95,1.3
1.8TFTSD = drill 1 square: P$1 55.58,8.5; P$9 2.76,14 | drill 1 octagon: P$2 55.58,11.04; P$3 55.58,13.58; P$4 55.58,16.12; P$5 55.58,18.66; P$6 55.58,21.2; P$7 55.58,23.74; P$8 55.58,26.28; P$10 2.76,16.54; P$11 2.76,19.08; P$12 2.76,21.62 | hole 2.8: 3,3; 3,31.5; 55,31.5; 55,3
GY-521 = drill 0.9 square: P$1 0,0 | drill 0.9 octagon: P$2 2.54,0; P$3 5.08,0; P$4 7.62,0; P$5 10.16,0; P$6 12.7,0; P$7 15.24,0; P$8 17.78,0 | hole 2.8: 0.635,12.7; 17.145,12.7
HMC5883L = drill 0.9 square: P$1 0,5.08 | drill 0.9 octagon: P$2 0,2.54; P$3 0,0; P$4 0,-2.54; P$5 0,-5.08
NRF24L01+ = drill 0.9 square: P$1 -1.016,1.016 | drill 0.9 octagon: P$2 -1.016,-1.524; P$3 -1.016,-4.064; P$4 -1.016,-6.604; P$5 1.524,-6.604; P$6 1.524,-4.064; P$7 1.524,-1.524; P$8 1.524,1.016
PNA460XM = drill 1.016 pad 1.93 square: 1 -2.54,0 | drill 1.016 pad 1.93: 2 0,0; 3 2.54,0
1X04 = drill 1.016 long: 1 -3.81,0; 2 -1.27,0; 3 1.27,0; 4 3.81,0
B5B-XH = drill 0.8 square: P$1 -5.08,0 | drill 0.8: P$2 -2.54,0; P$3 0,0; P$4 2.54,0; P$5 5.08,0

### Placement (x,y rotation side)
BATT  3.81,23.34 270 top
C1  124.71,42.39 90 top
C2  44.45,39.21 180 top
C3  128.91,52.04 270 top
C4  131.44,52.04 270 top
C5  22.86,46.83 0 top
C6  25.02,83.66 0 top
C7  63.5,22.07 270 top
C8  70.48,37.31 180 top
C9  69.85,54.13 0 top
C10  111.76,46.2 0 top
C11  65.72,22.07 270 top
C12  111.76,41.12 0 top
C13  111.76,63.98 90 top
C14  127.64,42.39 270 top
C15  130.3,70.33 0 top
C16  130.3,66.52 0 top
C17  26.99,31.91 270 top
C18  10.16,22.7 0 top
C19  25.4,27.15 180 top
C20  3.81,29.05 0 top
C21  10.16,25.88 180 top
C22  56.26,72.99 0 top
C23  61.34,72.99 180 top
CONN1  128.27,30.96 0 top
CONN2  125.73,79.22 180 top
CONN3  101.22,79.22 180 top
CONN4  100.33,76.68 180 top
CONN5  110.49,30.96 0 top
D2  6.99,61.12 90 top
D3  34.29,37.31 180 top
D4  3.81,32.23 0 top
D13  102.87,70.33 0 top
D13_2  44.45,46.83 0 top
F1  16.51,46.83 0 top
F2  16.51,83.66 0 top
FET1  149.86,48.74 0 top
FET3  22.86,32.54 0 top
JP1  34.29,57.63 270 top
JP2  151.13,53.82 90 top
JP3  134.62,58.89 270 top
JP4  94.61,15.24 0 top
L1  111.76,43.66 0 top
L2  24.13,36.67 0 top
MINIUSB  6.35,79.22 0 top
MINIUSB1  6.35,42.39 0 top
MUX  97.16,8.1 0 top
Q1  124.21,68.42 90 top
Q2  84.45,6.83 180 bottom
Q3  93.34,6.83 180 bottom
Q4  100.97,6.83 180 bottom
Q5  109.86,6.83 180 bottom
Q6  58.8,70.33 180 top
R1  84.45,10.24 180 bottom
R2  130.81,42.39 90 top
R3  84.45,3.41 0 bottom
R4  16.51,78.45 180 top
R5  16.51,80.74 180 top
R6  102.87,67.79 180 top
R7  10.16,69.06 180 top
R8  10.16,65.88 180 top
R9  107.95,51.15 180 top
R10  93.34,9.76 180 bottom
R11  93.34,3.41 0 bottom
R12  100.97,9.76 180 bottom
R13  100.97,3.41 0 bottom
R14  109.86,9.76 180 bottom
R15  109.86,3.41 0 bottom
R16  16.51,41.5 180 top
R17  10.16,32.23 180 top
R18  144.78,48.74 0 top
R19  10.16,29.05 180 top
R20  44.45,44.29 180 top
R21  10.16,56.36 180 top
R22  10.16,52.55 180 top
R23  30.48,46.2 90 top
R24  44.45,41.75 180 top
R25  16.51,44.04 180 top
R26  78.74,81.76 270 top
R27  82.55,81.76 270 top
R46  31.11,31.91 90 top
R49  34.92,31.91 90 top
R51  33.34,27.15 180 top
RX  3.81,69.06 0 top
RX1  3.81,56.36 0 top
S1  35.56,46.2 270 top
S2  135.89,46.7 270 top
SER_CPU2  36.83,70.33 90 top
SERVO1(USONIC)  143.51,56.36 90 top
SERVO2(GRIP)  143.51,74.14 90 top
SERVO3(GRIPROT)  143.51,36.04 90 top
SHIFT1  74HC595D  [SO16']  99.06,55.09 270 top
SHIFT2  74HC595D  [SO16']  99.06,43.66 270 top
STEPPER_DRIVER  88.9,55.09 90 top
TX  3.81,65.88 0 top
TX1  3.81,52.55 0 top
U1  119.38,55.09 180 top
U2  58.42,55.09 180 top
U3  58.42,22.38 270 top
U4  27.94,23.34 90 top
U5  16.83,33.18 90 top
U$2  39.37,84.04 270 top
U$3  40.64,86.84 0 top
U$4  67.31,86.84 90 top
U$5  41.91,22.07 0 top
U$10  21.59,55.09 270 top
ULTRASONIC  77.47,55.09 90 top
X1  78.74,39.85 90 top
X2  78.74,70.33 90 top

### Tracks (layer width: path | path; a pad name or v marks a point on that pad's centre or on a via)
2D13
  Top 0.305: 52.59,51.91 U2.32 51.41,51.89 50.8,51.28 50.8,47.15 47.94,44.29 R20.1
2D+  (via drill 0.3 pad 0.3)
  Top 0.254: U2.4 62.88,53.49 v62.23,54.13
  Top 0.305: v26.43,41.51 17.95,41.51 R16.1
  Bottom 0.254: v62.23,54.13 43.18,54.13
  Bottom 0.305: 43.18,54.13 30.56,41.51 v26.43,41.51
2D-  (via drill 0.3 pad 0.3)
  Top 0.305: U2.3 61.77,52.69 v61.59,52.86 | R25.1 v21.59,44.04
  Bottom 0.305: v61.59,52.86 60.96,53.5 43.5,53.5 30.48,40.48 25.15,40.48 v21.59,44.04
2MISO  (via drill 0.3 pad 0.3)
  Top 0.305: v50.8,60.17 v50.8,63.98 | v62.55,64.61 64.77,66.83 64.77,74.14 63.18,75.72 56.52,75.72 54.61,77.63 54.61,82.07 55.24,82.71 57.78,82.71 58.42,82.07 58.42,81.28 U$2.P$11 | v62.23,58.9 62.42,59.09 U2.11 | JP1.1 35.88,59.21 38.1,59.21 v40.48,56.83 41.91,55.4 v41.91,50.01
  Bottom 0.305: v40.48,56.83 60.17,56.83 v62.23,58.9 62.04,59.09 51.88,59.09 v50.8,60.17 | v50.8,63.98 51.44,64.61 v62.55,64.61 | U$5.P$4 38.1,18.26 38.1,46.2 v41.91,50.01
2MOSI  (via drill 0.3 pad 0.3)
  Top 0.254: 68.42,62.71 v68.42,60.33
  Top 0.305: v61.91,57.31 62.89,58.29 U2.10 64.25,58.26 v66.36,58.26 | SHIFT1.14 99.69,56.99 98.42,55.72 v98.42,53.5 98.42,50.32 97.16,49.05 94.3,49.05 91.76,46.51 v91.76,44.29 | U$2.P$10 55.91,79.19 58.42,76.68 63.5,76.68 66.04,74.14 66.04,65.09 68.42,62.71
  Bottom 0.254: JP1.4 37.47,56.04 60.64,56.04
  Bottom 0.305: U$5.P$6 50.11,18 U$2.P$6 65.29,33.18 88.27,33.18 91.76,36.67 v91.76,44.29 | 60.64,56.04 v61.91,57.31 | v98.42,53.5 98.11,53.18 85.72,53.18 78.58,60.33 v68.42,60.33 v66.36,58.26
2RESET  (via drill 0.3 pad 0.3)
  Top 0.305: R23.1 30.48,43.34 32.07,41.75 33.34,41.75 33.66,42.07 S1.4 S1.3 33.66,51.91 JP1.5 | U2.13 61.62,62.1 62.23,62.71 66.04,62.71 66.99,61.75 v66.99,60.33
  Bottom 0.305: v66.99,60.33 66.2,60.33 64.77,58.9 64.77,56.36 64.29,55.88 63.02,55.88 61.91,54.77 42.86,54.77 39.05,50.96 35.88,50.96 JP1.5
2RXLED  (via drill 0.3 pad 0.3)
  Top 0.305: U2.8 68.91,56.69 71.12,58.9 71.12,63.34 70.64,63.82 v69.85,63.82 | v52.39,63.82 49.21,66.99 43.97,66.99 38.89,61.91 22.54,61.91 16.99,56.36 R21.1
  Bottom 0.305: v69.85,63.82 v52.39,63.82
2SCK  (via drill 0.3 pad 0.3)
  Top 0.254: JP1.3 35.56,53.82 v40.64,53.82
  Top 0.305: SHIFT2.11 103.82,41.75 v104.14,42.07 | v103.82,53.18 SHIFT1.11 v99.69,53.18 | v62.71,56.83 63.36,57.49 U2.9 67.17,57.49 v67.31,57.63 | v92.87,32.23 101.6,32.23 104.14,34.77 104.14,38.58 v105.41,39.85 | U$2.P$12 60.99,80.46 66.67,74.77 66.67,65.56 69.85,62.39 69.85,60.17 v69.22,59.53
  Bottom 0.254: U$5.P$3 41.91,16.99 51.63,16.99
  Bottom 0.305: 51.63,16.99 U$2.P$7 66.87,32.23 v92.87,32.23 | v103.82,53.18 104.14,52.86 v104.14,42.07 105.41,40.8 v105.41,39.85 | v40.64,53.82 42.23,55.4 61.28,55.4 v62.71,56.83 | v67.31,57.63 v69.22,59.53 73.66,59.53 75.56,57.63 80.01,57.63 85.41,52.23 98.74,52.23 v99.69,53.18
2TXLED  (via drill 0.3 pad 0.3)
  Top 0.305: U2.22 54.42,62.9 49.53,67.79 43.18,67.79 38.1,62.71 21.59,62.71 v16.51,57.63 | v15.24,52.55 R22.1
  Bottom 0.305: v16.51,57.63 16.51,53.82 v15.24,52.55
2XTAL1
  Top 0.406: C22.1 54.86,71.49 Q6.1 58.42,67.93 U2.17
2XTAL2
  Top 0.406: C23.1 62.74,71.49 Q6.2 59.22,67.97 U2.16
3.3V
  Top 0.305: C11.1 C7.1 63.37,23.33 62.23,23.33 | U$2.P$8 65.65,23.47 C11.1 | CONN5.2 106.68,29.69 105.41,28.42 77.47,28.42 72.39,23.34 65.85,23.34 C11.1 | 62.23,23.33 U3.5 | U$5.P$8 50.42,23.08 53.34,20.16 60.96,20.16 61.59,20.8 61.59,22.7 62.23,23.33
A0
  Top 0.305: U1.36 116.98,38.44 121.92,33.5 CONN1.1
A1
  Top 0.305: U1.37 117.78,38.91 124.46,32.23 CONN1.2
A2
  Top 0.305: U1.38 118.58,39.38 124.46,33.5 125.73,33.5 127,32.23 CONN1.3
A3
  Top 0.305: U1.39 119.38,39.85 124.46,34.77 127,34.77 129.54,32.23 CONN1.4
A4
  Top 0.305: U1.40 120.18,40.32 124.46,36.04 128.27,36.04 132.08,32.23 CONN1.5
A5
  Top 0.305: U1.41 120.98,40.79 124.46,37.31 129.54,37.31 134.62,32.23 CONN1.6
AREF  (via drill 0.3 pad 0.3)
  Top 0.305: U1.42 121.78,45.07 123.19,43.66 | 123.19,43.66 124.58,43.66 C1.2 | CONN3.8 93.98,78.33 CONN4.8 99.06,71.6 99.06,66.52 105.41,60.17 105.41,56.36 107.95,53.82 v107.95,41.12 | v122.24,43.02 122.56,43.02 123.19,43.66 | U2.42 60.82,42.53 v63.5,39.85 66.04,37.31 C8.2 | v107.31,39.21 105.41,37.31 105.41,34.77 100.01,29.37 77.15,29.37 72.39,24.61 68.58,24.61 67.31,25.88 67.31,32.23 v63.5,36.04
  Bottom 0.254: v63.5,36.04 v63.5,39.85
  Bottom 0.305: v107.95,41.12 107.31,40.48 v107.31,39.21 107.79,38.74 109.38,38.74 112.08,41.43 120.65,41.43 v122.24,43.02
AVCC  (via drill 0.3 pad 0.3)
  Top 0.254: U1.24 114.8,58.29 115.09,58.58 117.16,58.58 118.11,57.63 v118.11,52.67
  Top 0.305: U1.44 v123.38,47.28 124.46,46.2 127,46.2 127.64,45.56 C14.1 | U1.24 112.37,58.29 111.76,58.9 C13.1 | U2.24 58.71,58.29 60.01,56.99 v60.01,52.71 | U2.44 62.42,46.7 v62.55,46.51 62.55,43.34 v64.77,41.12 | L1.2 v115.57,43.66 115.57,35.4 118.75,32.23 118.75,29.69 118.11,29.05 107.31,29.05 105.41,27.15 78.74,27.15 v77.47,25.88 | v66.04,30 v62.87,33.18
  Bottom 0.305: v123.38,47.28 119.76,43.66 v115.57,43.66 118.11,46.2 v118.11,52.67 | v60.01,52.71 60.01,51.7 U2.44 62.42,46.7 v62.55,46.51 | v77.47,25.88 70.17,25.88 v66.04,30 | v62.87,33.18 62.87,33.81 64.77,35.72 v64.77,41.12
D4  (via drill 0.3 pad 0.3)
  Top 0.254: v115.57,57.79 115.27,57.49 U1.25
  Top 0.305: CONN2.5 124.46,76.55 123.95,76.04 v120.27,76.04
  Bottom 0.254: 115.57,71.6 v115.57,57.79
  Bottom 0.305: v120.27,76.04 120.02,76.04 115.57,71.6
D5  (via drill 0.3 pad 0.3)
  Top 0.254: v116.84,57.79 116.84,53.82
  Top 0.305: U1.31 115.71,52.69 116.84,53.82
  Bottom 0.254: 116.84,67.79 v116.84,57.79
  Bottom 0.305: CONN2.6 121.92,72.87 116.84,67.79
D6
  Top 0.305: U1.27 112.23,55.89 109.22,58.9 109.22,69.06 CONN2.7
D7  (via drill 0.3 pad 0.3)
  Top 0.305: U1.1 125.18,49.29 v125.73,48.74 | v130.81,81.12 v128.14,81.12
  Bottom 0.305: v125.73,48.74 138.43,48.74 139.7,50.01 139.7,78.58 137.16,81.12 v130.81,81.12 | v128.14,81.12 118.75,81.12 CONN2.8
D8
  Top 0.305: CONN3.1 111.76,78.33 CONN4.1 111.76,75.41 107.95,71.6 107.95,58.9 111.76,55.09 U1.28
D9
  Top 0.305: CONN3.2 109.22,78.33 CONN4.2 109.22,74.01 107.31,72.1 107.31,58.52 111.54,54.29 U1.29
D10
  Top 0.305: CONN3.3 106.68,78.33 CONN4.3 106.68,58.13 111.33,53.49 U1.30
D11  (via drill 0.3 pad 0.3)
  Top 0.305: CONN4.4 104.14,78.33 CONN3.4 | U1.12 123.38,59.09 v123.19,58.9
  Bottom 0.254: 119.25,58.9 117.35,56.99 114.81,56.99 104.14,67.66
  Bottom 0.305: v123.19,58.9 119.25,58.9 | 104.14,67.66 CONN4.4
D12  (via drill 0.3 pad 0.3)
  Top 0.305: CONN4.5 101.6,78.33 CONN3.5 | U1.26 112.57,56.69 110.62,58.64 v110.62,60.17
  Bottom 0.305: CONN4.5 102.87,75.41 102.87,67.79 103,67.79 v110.62,60.17
D13
  Top 0.305: CONN3.6 99.06,78.33 CONN4.6 99.06,75.41 100.33,74.14 105.09,74.14 106.05,73.18 106.05,67.79 | U1.32 112.04,51.89 106.05,57.88 106.05,67.79 | R6.1 106.05,67.79
D+  (via drill 0.3 pad 0.3)
  Top 0.254: v123.51,53.5 125.17,53.5 U1.4
  Top 0.305: v28.89,64.93 17.93,75.89 R4.1
  Bottom 0.254: 119.38,55.09 85.72,55.09
  Bottom 0.305: v123.51,53.5 120.97,53.5 119.38,55.09 | 85.72,55.09 79.06,61.75 41.59,61.75 38.42,64.93 v28.89,64.93
D-  (via drill 0.3 pad 0.3)
  Top 0.305: U1.3 v122.87,52.69 | 18,80.8 arc90 R5.1 18.19,80.49 20.32,80.49 v36.83,63.98
  Bottom 0.254: 119.06,54.45 85.41,54.45 | 78.74,61.12 41.27,61.12
  Bottom 0.305: v122.87,52.69 120.83,52.69 119.06,54.45 | 85.41,54.45 78.74,61.12 | 41.27,61.12 38.42,63.98 v36.83,63.98
ECHO  (via drill 0.3 pad 0.3)
  Top 0.305: ULTRASONIC.2 74.93,53.82 v66.04,44.93 | v56.83,46.2 56.83,49.27 U2.37
  Bottom 0.305: v66.04,44.93 58.42,44.93 v56.83,46.2
GND  (via drill 0.3 pad 0.3)
  Top 0.305: v113.67,60.8 114.3,60.17
  other vias: 81.92,54.45 100.01,44.29 57.15,52.7 113.03,69.06 114.3,76.68 121.92,63.34 97.79,75.41 100.33,75.41 105.41,75.41 87.63,65.25 95.25,65.25 88.9,66.52 90.17,67.79 93.98,66.52 92.71,67.79 91.44,69.06 90.17,65.25 92.71,65.25 91.44,66.52 74.93,30.64 81.28,30.64 90.17,30.64 93.66,36.35 86.36,38.58 86.36,39.85 87.63,41.12 88.9,39.85 88.9,38.58 83.82,38.58 83.82,39.85 85.09,41.12 65.41,43.02 97.79,30.64 97.79,25.56 88.9,25.56 61.59,47.47 61.28,37.31 51.44,41.75 50.01,44.61 48.26,47.47 60.8,66.99 63.34,68.58 70.33,65.56 90.17,70.33 92.71,70.33 88.9,71.6 93.98,71.6 87.63,72.87 91.44,71.6 95.25,72.87 90.17,72.87 92.71,72.87
  pour Top (isolate 0.254): -1.27,105.89 156.21,103.35 156.21,8.1 -1.27,4.29
  pour Bottom (isolate 0.254): 77.47,103.35 77.47,88.11 142.24,88.11 149.86,81.76 156.21,81.76 156.21,29.69 149.86,29.69 142.24,22.07 77.47,22.07 77.47,6.83 35.56,6.83 35.56,18.26 0,18.26 0,91.92 35.56,91.92 35.56,103.35
IR
  Top 0.305: U$10.1 24.13,60.17 38.5,60.17 39.45,59.21 49.93,59.21 51.65,57.49 U2.25
IR_GND  (1 unrouted)
  Top 0.203: MUX.8 102.87,6.57 102.87,14.61 JP4.6
  Top 0.305: MUX.8 MUX.7 MUX.6
  Bottom 0.305: Q2.4 84.31,7.73 Q2.2 88,7.73 89.8,5.93 Q3.4 93.19,7.73 Q3.2 96.25,7.73 98.06,5.93 Q4.4 100.06,5.93 101.86,7.73 Q4.2 104.51,7.73 106.31,5.93 Q5.4 109.7,7.73 Q5.2
IR_OUT  (via drill 0.3 pad 0.3)
  Top 0.305: MUX.3 95.25,4.29 95.57,3.97 102.87,3.97 103.98,5.08 v103.98,13.89
  Bottom 0.203: JP4.4 98.42,16.51 101.92,16.51 103.98,14.45 v103.98,13.89
IR_VCC  (via drill 0.3 pad 0.3)
  Top 0.305: MUX.16 v92.71,12.38
  Bottom 0.305: 85.72,10.79 R1.2 | 97.95,1.27 104.3,1.27 106.44,3.41 R15.2 | 97.95,1.27 89.53,1.27 | 89.53,1.27 83.74,1.27 83.03,1.98 R3.2 81.52,3.41 80.64,4.29 80.64,11.27 81.68,12.3 84.93,12.3 85.88,11.36 R1.2 | R11.2 89.93,3.41 89.53,3.02 89.53,1.27 | R13.2 98.35,3.41 97.95,3.02 97.95,1.27 | v92.71,12.38 92.87,12.54 | R1.2 88.02,12.38 v92.71,12.38 | R14.2 111.28,11.04 110.97,11.35 102.23,11.35 | 102.23,11.35 94.61,11.35 | 94.61,11.35 93.74,11.35 v92.71,12.38 | R10.2 94.77,11.2 94.61,11.35 | R12.2 102.39,11.2 102.23,11.35 | JP4.2 92.71,15.88 v92.71,12.38
IRA
  Top 0.203: JP4.1 96.84,13.02 98.19,13.02 99.06,12.14 MUX.11
IRB
  Top 0.203: JP4.3 100.33,12.07 MUX.10
IRC
  Top 0.203: JP4.5 101.6,13.34 MUX.9
MISO
  Top 0.254: JP3.1 134.42,59.09 U1.11
MOSI
  Top 0.203: U1.10 132.69,58.29 133.35,57.63 135.89,57.63 135.89,57.62 JP3.4
MUX0  (via drill 0.3 pad 0.3)
  Top 0.305: v87.63,3.02 87,3.65 87,12.14 88.5,13.65 94.85,13.65 96.52,11.99 MUX.13
  Bottom 0.305: R3.1 86.41,3.54 Q2.3 86.36,5.88 86.36,2.7 86.68,3.02 v87.63,3.02
MUX1  (via drill 0.3 pad 0.3)
  Top 0.305: v96.68,2.22 91.28,2.22 88.58,4.92 88.58,12.38 89.3,13.1 94.38,13.1 95.25,12.22 MUX.14
  Bottom 0.305: 95.25,5.88 Q3.3 95.3,3.54 R11.1 95.81,3.02 v96.68,2.22
MUX2  (via drill 0.3 pad 0.3)
  Top 0.305: MUX.15 93.98,8.73 91.52,6.27 91.52,4.13 92.39,3.25 v104.46,3.25
  Bottom 0.305: 102.23,3.02 102.92,3.7 Q4.3 102.92,3.54 R13.1 102.55,3.25 v104.46,3.25
MUX3  (via drill 0.3 pad 0.3)
  Top 0.305: v97.79,12.22 MUX.12
  Bottom 0.305: R15.1 111.81,3.54 Q5.3 112.77,5.93 113.67,6.83 113.67,10.8 111.6,12.86 98.42,12.86 v97.79,12.22
MUX_OUT  (via drill 0.3 pad 0.3)
  Top 0.305: v102.23,37.31 98.42,33.5 92.71,33.5 91.44,32.23 68.58,32.23 60.02,40.79 U2.41
  Bottom 0.254: 110.49,37.31 v102.23,37.31
  Bottom 0.305: JP2.4 146.05,53.82 146.05,52.55 133.35,39.85 113.03,39.85 110.49,37.31
N$1
  Top 0.406: TX.C R8.2
N$2
  Top 0.406: MINIUSB.2 12.7,80.02 13.42,80.74 R5.2
N$3
  Top 0.305: U2.21 55.22,63.37 49.53,69.06 SER_CPU2.1
N$4
  Top 0.305: U2.20 56.02,63.84 48.26,71.6 SER_CPU2.2
N$5
  Top 0.406: MINIUSB.3 12.7,79.22 13.46,78.45 R4.2
N$6
  Top 0.305: R9.1 113.54,51.12 U1.33
N$7
  Top 0.406: D13.A R6.2
N$8
  Top 0.305: U2.6 66.04,55.09 66.99,54.13 C9.1
N$9
  Top 0.406: R7.2 RX.C
N$10
  Bottom 0.305: Q2.1 83.03,8.25 R1.1
N$11
  Bottom 0.305: Q3.1 91.92,8.25 R10.1
N$12
  Bottom 0.305: Q4.1 99.54,8.25 R12.1
N$13
  Top 0.406: MINIUSB.1 11.76,80.82 12.7,81.76 12.7,83.03 13.34,83.66 F2.1
N$14
  Bottom 0.305: Q5.1 108.43,8.25 R14.1
N$15
  Top 0.305: U1.6 128.4,55.09 128.91,54.58 C3.1
N$16
  Top 0.305: R18.2 148.59,48.74 148.91,48.42 FET1.1
N$17
  Top 0.305: U2.33 52.62,45.48 48.9,41.75 R24.1
N$18
  Top 0.406: F1.1 13.34,46.83 12.7,46.2 12.7,45.18 11.51,43.99 MINIUSB1.1
N$19
  Top 0.305: FET3.1 21.91,22.06 22.54,21.43 27.94,21.43 28.89,22.38 U4.1
N$20
  Top 0.305: U5.5 14.61,32.23 13.34,30.96 13.34,29.69 12.7,29.05 R19.1
N$21
  Top 0.305: U5.1 17.46,32.23 16.51,33.18 13.65,33.18 12.7,32.23 R17.1
N$22
  Top 0.305: D4.C R17.2
N$23
  Top 0.305: U4.4 31.48,24.34 32.07,24.92 32.07,26.99 R51.2 31.92,28.58 32.38,29.05 34.61,29.05 34.92,29.37 R49.1
N$24
  Top 0.305: D3.A 25.53,36.51 L2.2 25.4,36.54 25.4,35.08 23.86,33.54 FET3.3
N$25
  Top 0.305: U4.8 27.62,22.39 28.26,23.02 | 28.26,23.02 28.93,23.69 U4.3 | U4.5 26.67,24.34 | 26.67,24.34 26.94,24.34 28.26,23.02 | 26.67,24.34 26.8,24.47 C19.1 28.89,27.15 31.11,29.37 R46.1
N$26
  Top 0.305: X2.P$4 82.55,69.06 82.55,61.44 85.09,58.9 STEPPER_DRIVER.11
N$27
  Top 0.305: X2.P$3 81.92,67.15 81.92,60.8 85.09,57.63 STEPPER_DRIVER.12
N$28
  Top 0.305: X2.P$2 81.28,65.25 81.28,60.17 85.09,56.36 STEPPER_DRIVER.13
N$29
  Top 0.305: X2.P$1 80.64,63.34 80.64,59.53 85.09,55.09 STEPPER_DRIVER.14
N$30
  Top 0.305: X1.P$4 80.64,44.29 80.64,49.37 85.09,53.82 STEPPER_DRIVER.15
N$31
  Top 0.305: X1.P$3 81.28,42.39 81.28,48.74 85.09,52.55 STEPPER_DRIVER.16
N$32
  Top 0.305: X1.P$2 81.92,40.48 81.92,48.1 85.09,51.28 STEPPER_DRIVER.17
N$33
  Top 0.305: X1.P$1 82.55,38.58 82.55,47.47 85.09,50.01 STEPPER_DRIVER.18
N$34
  Top 0.305: R20.2 43.03,46.75 D13_2.A
N$35
  Top 0.406: TX1.C R22.2
N$36
  Top 0.406: RX1.C R21.2
N$37
  Top 0.305: MINIUSB1.2 12.74,43.19 13.59,44.04 R25.2
N$38
  Top 0.305: MINIUSB1.3 12.7,42.39 13.59,41.5 R16.2
N$41  (via drill 0.3 pad 0.3)
  Top 0.305: SHIFT2.15 v100.01,46.83
  Bottom 0.254: 110.49,36.35 101.28,36.35 99.06,38.58
  Bottom 0.305: JP2.1 148.59,51.28 145.73,51.28 133.67,39.21 113.35,39.21 110.49,36.35 | v100.01,46.83 99.06,45.88 99.06,38.58
N$42  (via drill 0.3 pad 0.3)
  Top 0.305: v97.79,48.1 SHIFT2.1
  Bottom 0.254: 110.81,35.72 100.97,35.72 98.5,38.18 98.5,47.39 v97.79,48.1
  Bottom 0.305: JP2.3 153.03,54.45 153.03,53.18 150.5,50.64 146.05,50.64 133.99,38.58 113.67,38.58 110.81,35.72
N$43  (via drill 0.3 pad 0.3)
  Top 0.305: v151.76,50.64 153.03,51.91 153.03,57.94 152.08,58.9 JP2.5 | SHIFT2.2 v97.79,46.83
  Bottom 0.254: 111.12,34.77 100.33,34.77 97.79,37.31
  Bottom 0.305: 111.12,34.77 113.98,37.62 134.3,37.62 146.69,50.01 151.13,50.01 v151.76,50.64 | v97.79,46.83 97.79,37.31
N$44  (via drill 0.3 pad 0.3)
  other vias: 133.35,77.95
N$45
  Top 0.254: FET1.3 149.86,57.63 JP2.6
NRF_CE  (via drill 0.3 pad 0.3)
  Top 0.305: v47.78,52.07 50,54.29 U2.29
  Bottom 0.305: U$5.P$2 38.73,22.7 38.73,43.02 v47.78,52.07
NRF_CSN  (via drill 0.3 pad 0.3)
  Top 0.305: v49.05,52.07 50.47,53.49 U2.30
  Bottom 0.305: U$5.P$7 42.23,21.75 42.23,24.29 39.37,27.15 39.37,42.39 v49.05,52.07
NRF_IRQ  (via drill 0.3 pad 0.3)
  Top 0.305: U$5.P$5 47.5,19.53 v49.53,19.53 | v67.31,50.01 66.23,51.09 U2.1
  Bottom 0.305: v67.31,50.01 67.31,36.67 61.91,30.96 58.74,30.96 56.83,29.05 56.83,26.83 v49.53,19.53
RESET  (via drill 0.3 pad 0.3)
  Top 0.305: U1.13 122.58,62.1 123.19,62.71 125.73,62.71 v127,61.44 | v133.22,55.09 133.34,55.09 JP3.5 133.99,53.18 S2.3 v133.99,46.83 S2.4 133.99,41.5 133.45,40.96 R2.1 | v108.46,39.85 108.46,34 107.95,33.5 105.41,33.5 104.14,32.23 CONN5.1
  Bottom 0.305: v127,61.44 130.18,58.26 130.18,55.85 130.94,55.09 v133.22,55.09 | v133.99,46.83 124.21,46.83 119.76,42.39 111,42.39 v108.46,39.85
RX-I
  Top 0.305: CONN2.1 134.62,76.68 132.08,74.14 123.19,74.14 116.98,67.93 U1.20
RXLED  (via drill 0.3 pad 0.3)
  Top 0.305: U1.8 122.89,56.69 v122.87,56.67 | v13.97,69.06 R7.1 11.43,69.06
  Bottom 0.254: 119.38,55.72 86.04,55.72
  Bottom 0.305: v122.87,56.67 120.33,56.67 119.38,55.72 | 86.04,55.72 79.38,62.39 42.23,62.39 38.1,66.52 19.05,66.52 16.51,69.06 v13.97,69.06
S1
  Top 0.254: SHIFT1.15 99.95,58.26 97.54,60.67 94.61,60.67 92.84,58.9 STEPPER_DRIVER.8
S1OVERFLOW
  Top 0.305: SHIFT2.14 103.5,45.56 104.14,46.2 104.14,50.01 103.5,50.64 SHIFT1.9
S2
  Top 0.254: STEPPER_DRIVER.7 92.71,57.63 94.61,59.53 SHIFT1.1
S2O4  (via drill 0.3 pad 0.3)
  Top 0.305: R18.1 142.24,48.74 139.7,46.2 v139.7,41.12 | v94.3,45.56 SHIFT2.3
  Bottom 0.254: 111.44,33.81 100.01,33.81 93.34,40.48
  Bottom 0.305: v139.7,41.12 135.25,36.67 114.3,36.67 111.44,33.81 | 93.34,40.48 93.34,44.61 v94.3,45.56
S3
  Top 0.254: STEPPER_DRIVER.6 92.71,56.36 94.61,58.26 SHIFT1.2
S4
  Top 0.254: STEPPER_DRIVER.5 92.71,55.09 94.61,56.99 SHIFT1.3
S5
  Top 0.254: STEPPER_DRIVER.4 92.71,53.82 94.61,55.72 SHIFT1.4
S6
  Top 0.254: STEPPER_DRIVER.3 92.71,52.55 94.61,54.45 SHIFT1.5
S7
  Top 0.254: STEPPER_DRIVER.2 92.71,51.28 94.61,53.18 SHIFT1.6
S8
  Top 0.254: STEPPER_DRIVER.1 92.71,50.01 94.61,51.91 SHIFT1.7
S_GRIP  (via drill 0.3 pad 0.3)
  Top 0.305: v89.22,81.44 90.49,82.71 134.62,82.71 140.65,76.68 SERVO2(GRIP).3 | v87.63,79.85 85.09,79.85 v80.33,75.09 | v48.9,65.25 48.26,64.61 v48.26,60.17 | U2.27 48.73,55.89 48.26,56.36 v48.26,57.63
  Bottom 0.305: v89.22,81.44 v87.63,79.85 | v80.33,75.09 79.38,74.14 76.2,74.14 68.58,66.52 62.23,66.52 60.96,65.25 v48.9,65.25 | v48.26,57.63 v48.26,60.17
S_GRIPROT  (via drill 0.3 pad 0.3)
  Top 0.305: U2.12 65.32,60.89 v68.58,57.63
  Bottom 0.254: 111.76,33.18 99.69,33.18 92.71,40.16
  Bottom 0.305: SERVO3(GRIPROT).3 138.43,38.58 135.89,36.04 114.62,36.04 111.76,33.18 | 92.71,40.16 92.71,46.2 87.63,51.28 85.09,51.28 82.55,48.74 76.2,48.74 73.66,51.28 73.66,55.09 71.12,57.63 v68.58,57.63
S_USONIC  (via drill 0.3 pad 0.3)
  Top 0.305: v101.44,38.1 97.47,34.13 92.08,34.13 91.12,33.18 68.9,33.18 v60.96,41.12 | v54.61,52.55 54.47,52.69 U2.31
  Bottom 0.254: 110.33,38.1 v101.44,38.1
  Bottom 0.305: SERVO1(USONIC).3 141.6,58.9 140.97,58.26 140.97,48.42 133.03,40.48 112.71,40.48 110.33,38.1 | v60.96,41.12 58.42,41.12 54.61,44.93 v54.61,52.55
SCK
  Top 0.305: JP3.3 133.35,56.36 132.22,57.49 U1.9
SCL  (via drill 0.3 pad 0.3)
  Top 0.305: CONN3.10 88.9,78.33 CONN4.10 | U1.18 v118.58,67.37 | CONN3.10 91.57,80.99 126.11,80.99 127,80.11 CONN2.4 | CONN3.10 87.25,81.76 79.38,81.76 78.74,82.39 R26.1 78.74,84.3 78.11,84.93 69.22,84.93 U$4.P$3 | U2.18 57.62,64.78 45.72,76.68 U$3.P$3
  Bottom 0.305: CONN2.4 127,75.79 v118.58,67.37 | U$4.P$3 66.04,88.11 46.99,88.11 U$3.P$3
SD_CS  (via drill 0.3 pad 0.3)
  Top 0.305: v46.99,64.61 v46.99,60.17 | v46.99,57.63 46.99,56.36 48.26,55.09 U2.28
  Bottom 0.305: U$2.P$9 53.37,71.57 54.61,70.33 54.61,67.79 53.34,66.52 48.26,66.52 46.99,65.25 v46.99,64.61 | v46.99,60.17 v46.99,57.63
SDA  (via drill 0.3 pad 0.3)
  Top 0.305: U1.19 v117.78,64.99 | CONN3.9 91.44,78.33 CONN4.9 | v88.91,83.18 R27.1 82.55,84.3 81.28,85.57 71.12,85.57 U$4.P$4 68.58,88.11 49.53,88.11 U$3.P$4 46.99,85.57 v46.99,83.03 | U2.19 56.82,64.31 v53.34,67.79
  Bottom 0.305: v117.78,64.99 117.86,64.99 129.54,76.68 CONN2.3 129.54,81.12 128.27,82.39 115.32,82.39 113.92,80.99 94.11,80.99 CONN3.9 92.39,79.28 92.39,82.87 92.08,83.18 v88.91,83.18 | v53.34,67.79 53.34,70.33 46.99,76.68 v46.99,83.03
SHIFT_RCK  (via drill 0.3 pad 0.3)
  Top 0.305: SHIFT1.12 104.14,54.45 104.78,53.82 104.78,43.66 104.14,43.02 SHIFT2.12 100.65,43.02 100.33,42.7 v100.33,41.75 | U2.26 50.47,56.69 48.58,58.58 45.72,58.58 44.45,57.31 44.45,31.27 45.72,30 v45.72,26.51 | v48.9,21.43 50.16,21.43 53.34,18.26 68.58,18.26 v77.47,27.15 | v100.33,39.21 v96.2,35.08
  Bottom 0.305: v45.72,26.51 45.72,24.61 v48.9,21.43 | v100.33,41.75 v100.33,39.21 | v96.2,35.08 93.98,32.86 93.98,28.42 92.71,27.15 v77.47,27.15
TFT_CS  (via drill 0.3 pad 0.3)
  Top 0.305: U2.40 v59.22,33.66
  Bottom 0.305: v59.22,33.66 58.74,33.18 57.15,33.18 52.95,28.98 U$2.P$3
TFT_DC
  Top 0.305: U2.38 57.62,31.12 58.1,30.64 58.1,28.54 U$2.P$5
TFT_RST  (via drill 0.3 pad 0.3)
  Top 0.305: U2.39 v58.42,32.23
  Bottom 0.305: v58.42,32.23 55.49,29.3 U$2.P$4
TRIG  (via drill 0.3 pad 0.3)
  Top 0.305: ULTRASONIC.3 76.2,56.36 v63.5,43.66 | v56.2,45.24 56.02,45.42 U2.36
  Bottom 0.305: v63.5,43.66 57.78,43.66 v56.2,45.24
TX-O
  Top 0.305: CONN2.2 132.08,76.68 130.81,75.41 123.19,75.41 116.18,68.4 U1.21
TXLED  (via drill 0.3 pad 0.3)
  Top 0.254: v119.38,56.99 119.38,57.63
  Top 0.305: U1.22 115.38,59.4 115.57,59.21 117.79,59.21 119.38,57.63 | v12.7,71.6 11.43,71.6 10.16,70.33 10.16,66.52 10.79,65.88 R8.1
  Bottom 0.254: 86.36,56.36 118.75,56.36 v119.38,56.99
  Bottom 0.305: 86.36,56.36 79.69,63.02 42.55,63.02 38.42,67.15 21.27,67.15 16.83,71.6 v12.7,71.6
USB1_VIN  (via drill 0.3 pad 0.3)
  Top 0.305: C6.1 v20.95,83.66 F2.2 | v10.16,63.98 10.16,62.71 9.53,62.07 D2.2
  Bottom 0.305: v20.95,83.66 17.14,83.66 16.51,83.03 16.51,75.41 15.24,74.14 11.43,74.14 10.16,72.87 v10.16,63.98
USB2_VIN  (via drill 0.3 pad 0.3)
  Top 0.305: D2.1 9.52,60.17 10.16,59.53 v10.16,58.1 | F1.2 18.24,46.91 v19.76,46.91 19.84,46.83 C5.1
  Bottom 0.305: v10.16,58.1 10.16,50.01 11.43,48.74 19.05,48.74 19.76,48.02 v19.76,46.91
USB_VIN  (via drill 0.3 pad 0.3)
  Top 0.305: D4.A 2.41,32.13 | 2.41,32.13 C20.1 | D2.3 v4.13,61.12 | U5.4 4.45,34.13 v3.81,34.77 3.81,34.45 2.54,33.18 2.54,32.26 2.41,32.13
  Bottom 0.305: v4.13,61.12 3.49,61.12 2.54,60.17 2.54,36.04 v3.81,34.77
VBATT  (via drill 0.3 pad 0.3)
  Top 0.305: BATT.2 4.8,20.8 10.79,20.8 11.56,21.56 C18.2 C21.1 12.7,25.88 14.61,27.78 14.61,30.32 15.24,30.96 v15.88,30.96 | v16.83,34.13 17.46,34.13 U5.3 | U5.3 | U5.3 19.68,34.13 20.32,34.77 20.32,36.04 20.95,36.67 L2.1
  Bottom 0.305: v15.88,30.96 16.83,31.91 v16.83,34.13
VCC  (via drill 0.3 pad 0.3)  (1 unrouted)
  Top 0.305: U1.7 125.22,55.85 | 131.44,54.58 C4.1 | 110.36,46.07 110.49,46.2 | 110.49,46.33 C10.1 | RX1.A TX.A | C17.1 31.09,33.31 R46.2 R49.2 34.92,36.51 D3.C | U3.3 55.88,21.43 55.88,23.34 U3.1 51.76,23.33 47.87,27.22 U$2.P$1 47.87,30.08 45.85,32.1 v45.85,37.44 | R26.2 R27.2 | R26.2 X2.P$5 | R26.2 76.35,80.33 72.39,84.3 63.5,84.3 62.23,85.57 U$4.P$1 | X2.P$5 83.82,70.33 83.82,61.44 85.09,60.17 STEPPER_DRIVER.10 88.9,60.17 90.17,61.44 97.79,61.44 99.69,59.53 SHIFT1.16 | X1.P$5 80.01,46.2 80.01,57.94 79.06,58.9 ULTRASONIC.4 75.88,58.9 | 75.88,58.9 75.25,59.53 75.25,62.39 76.83,63.98 76.83,73.5 X2.P$5 | SHIFT1.10 100.01,51.91 99.06,50.96 99.06,48.1 | 99.06,48.1 99.06,41.12 99.69,40.48 SHIFT2.10 104.14,40.48 106.36,42.7 v106.36,46.2 | SHIFT2.16 99.06,48.1 | JP3.2 139.69,56.36 SERVO1(USONIC).2 146.05,56.36 | 146.05,56.36 JP2.2 144.78,50.01 144.78,47.47 146.05,46.2 146.05,36.67 145.41,36.04 SERVO3(GRIPROT).2 | 146.05,56.36 146.69,56.99 146.69,72.87 145.41,74.14 SERVO2(GRIP).2 | 60.82,51.89 55.54,51.89 54.42,50.77 U2.34 54.42,41.88 51.75,39.21 C2.1 v45.85,37.44 | 60.82,51.89 U2.2 | U2.14 60.82,55.89 | 60.82,55.89 60.82,51.89 | 60.82,55.89 U2.7 72.87,55.89 75.88,58.9 | R23.2 30.33,47.47 | v30.48,50.01 R23.2 | v45.85,37.44 45.72,37.31 | D3.C 41.11,36.51 v41.91,37.31 | D3.C 33.29,38.31 27.94,43.66 27.94,46.91 28.65,47.63 R23.2 | TX1.A 2.31,51.51 3.81,50.01 19.05,50.01 U$10.3
  Top 0.406: TX.A RX.A | 131.44,54.58 130.18,55.85 125.22,55.85 121.78,55.85 | 121.78,51.89 116.81,51.89 115.38,50.45 U1.34 112.31,49.29 v111.76,48.74 110.49,47.47 110.49,46.33 | 121.78,51.89 U1.2 126.39,51.89 127,51.28 127,49.37 130.81,45.56 R2.2 | U1.14 121.78,55.85 | 121.78,55.85 121.78,51.89 | v131.44,56.36 C4.1 | 110.36,46.07 L1.1 C12.1 110.36,33.37 109.22,32.23 CONN5.3 | RX1.A TX1.A
  Bottom 0.254: JP1.2 35.56,56.36 33.02,56.36 30.48,53.82
  Bottom 0.305: U$4.P$1 62.23,85.57 61.59,84.93 41.27,84.93 40.64,85.57 U$3.P$1 | v106.36,46.2 108.9,48.74 v111.76,48.74 | X2.P$5 87.63,84.3 135.89,84.3 140.97,79.22 140.97,74.61 141.45,74.14 SERVO2(GRIP).2 | 30.48,53.82 v30.48,50.01 27.94,52.55 U$10.3 | v41.91,37.31 45.72,37.31 v45.85,37.44
  Bottom 0.406: JP3.2 135.25,60.8 132.72,60.8 131.44,59.53 v131.44,56.36
XTAL1
  Top 0.406: Q1.1 124.21,70.33 | 124.21,70.33 C15.1 | U1.17 119.38,66.9 122.81,70.33 124.21,70.33
XTAL2
  Top 0.406: C16.1 124.21,66.52 Q1.2 123.81,65.25 121.92,65.25 120.18,63.51 U1.16

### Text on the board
Top: EDUBOT V0.1 BY / SEBASTIAN MUSZYTOWSKI | USER

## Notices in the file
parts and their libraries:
SparkFun-Connectors: Licensing: Creative Commons ShareAlike 4.0 International - https://creativecommons.org/licenses/by-sa/4.0
